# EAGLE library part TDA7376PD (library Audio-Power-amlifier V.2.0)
2 X 35W POWER AMPLIFIER FOR CAR RADIO
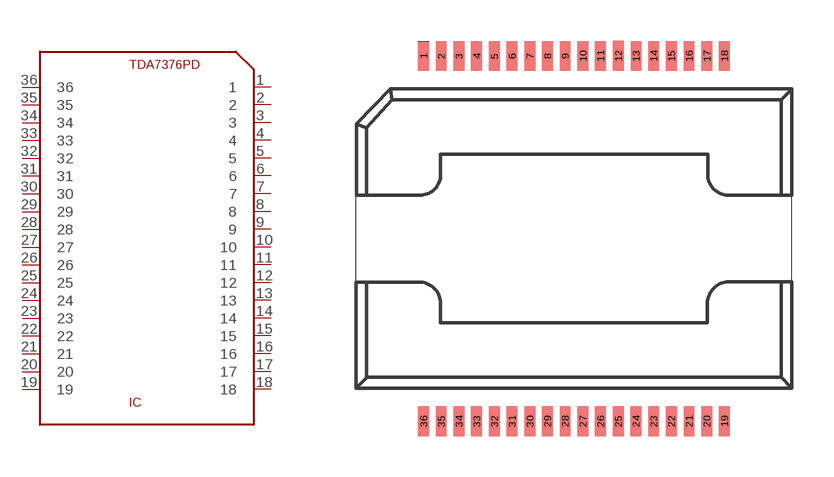
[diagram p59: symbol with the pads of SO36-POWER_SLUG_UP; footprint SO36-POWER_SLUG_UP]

Designator prefix IC

## TDA7376PD  [SO36-POWER_SLUG_UP]
1  1
2  2  pwr
3  3  pwr
4  4  nc
5  5  out
6  6  out
7  7  nc
8  8  out
9  9  out
10  10  pwr
11  11  pwr
12  12  in
13  13  in
14  14  nc
15  15  nc
16  16
17  17
18  18  pwr
19  19  nc
20  20
21  21  out
22  22  nc
23  23  nc
24  24  in
25  25  in
26  26  pwr
27  27  pwr
28  28  out
29  29  out
30  30  nc
31  31  out
32  32  out
33  33  out
34  34  pwr
35  35  pwr
36  36  nc

## Footprint SO36-POWER_SLUG_UP (pad centres in mm)
smd 0.4 x 1.1: 1 -5.525,6.7; 2 -4.875,6.7; 3 -4.225,6.7; 4 -3.575,6.7; 5 -2.925,6.7; 6 -2.275,6.7; 7 -1.62,6.7; 8 -0.975,6.7; 9 -0.325,6.7; 10 0.33,6.7; 11 0.975,6.7; 12 1.63,6.705; 13 2.28,6.7; 14 2.925,6.7; 15 3.575,6.7; 16 4.225,6.7; 17 4.88,6.7; 18 5.525,6.7; 19 5.525,-6.7; 20 4.875,-6.7; 21 4.225,-6.7; 22 3.575,-6.7; 23 2.925,-6.7; 24 2.275,-6.7; 25 1.625,-6.7; 26 0.975,-6.7; 27 0.325,-6.7; 28 -0.325,-6.7; 29 -0.975,-6.7; 30 -1.62,-6.7; 31 -2.275,-6.7; 32 -2.925,-6.7; 33 -3.575,-6.7; 34 -4.225,-6.7; 35 -4.875,-6.7; 36 -5.525,-6.7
